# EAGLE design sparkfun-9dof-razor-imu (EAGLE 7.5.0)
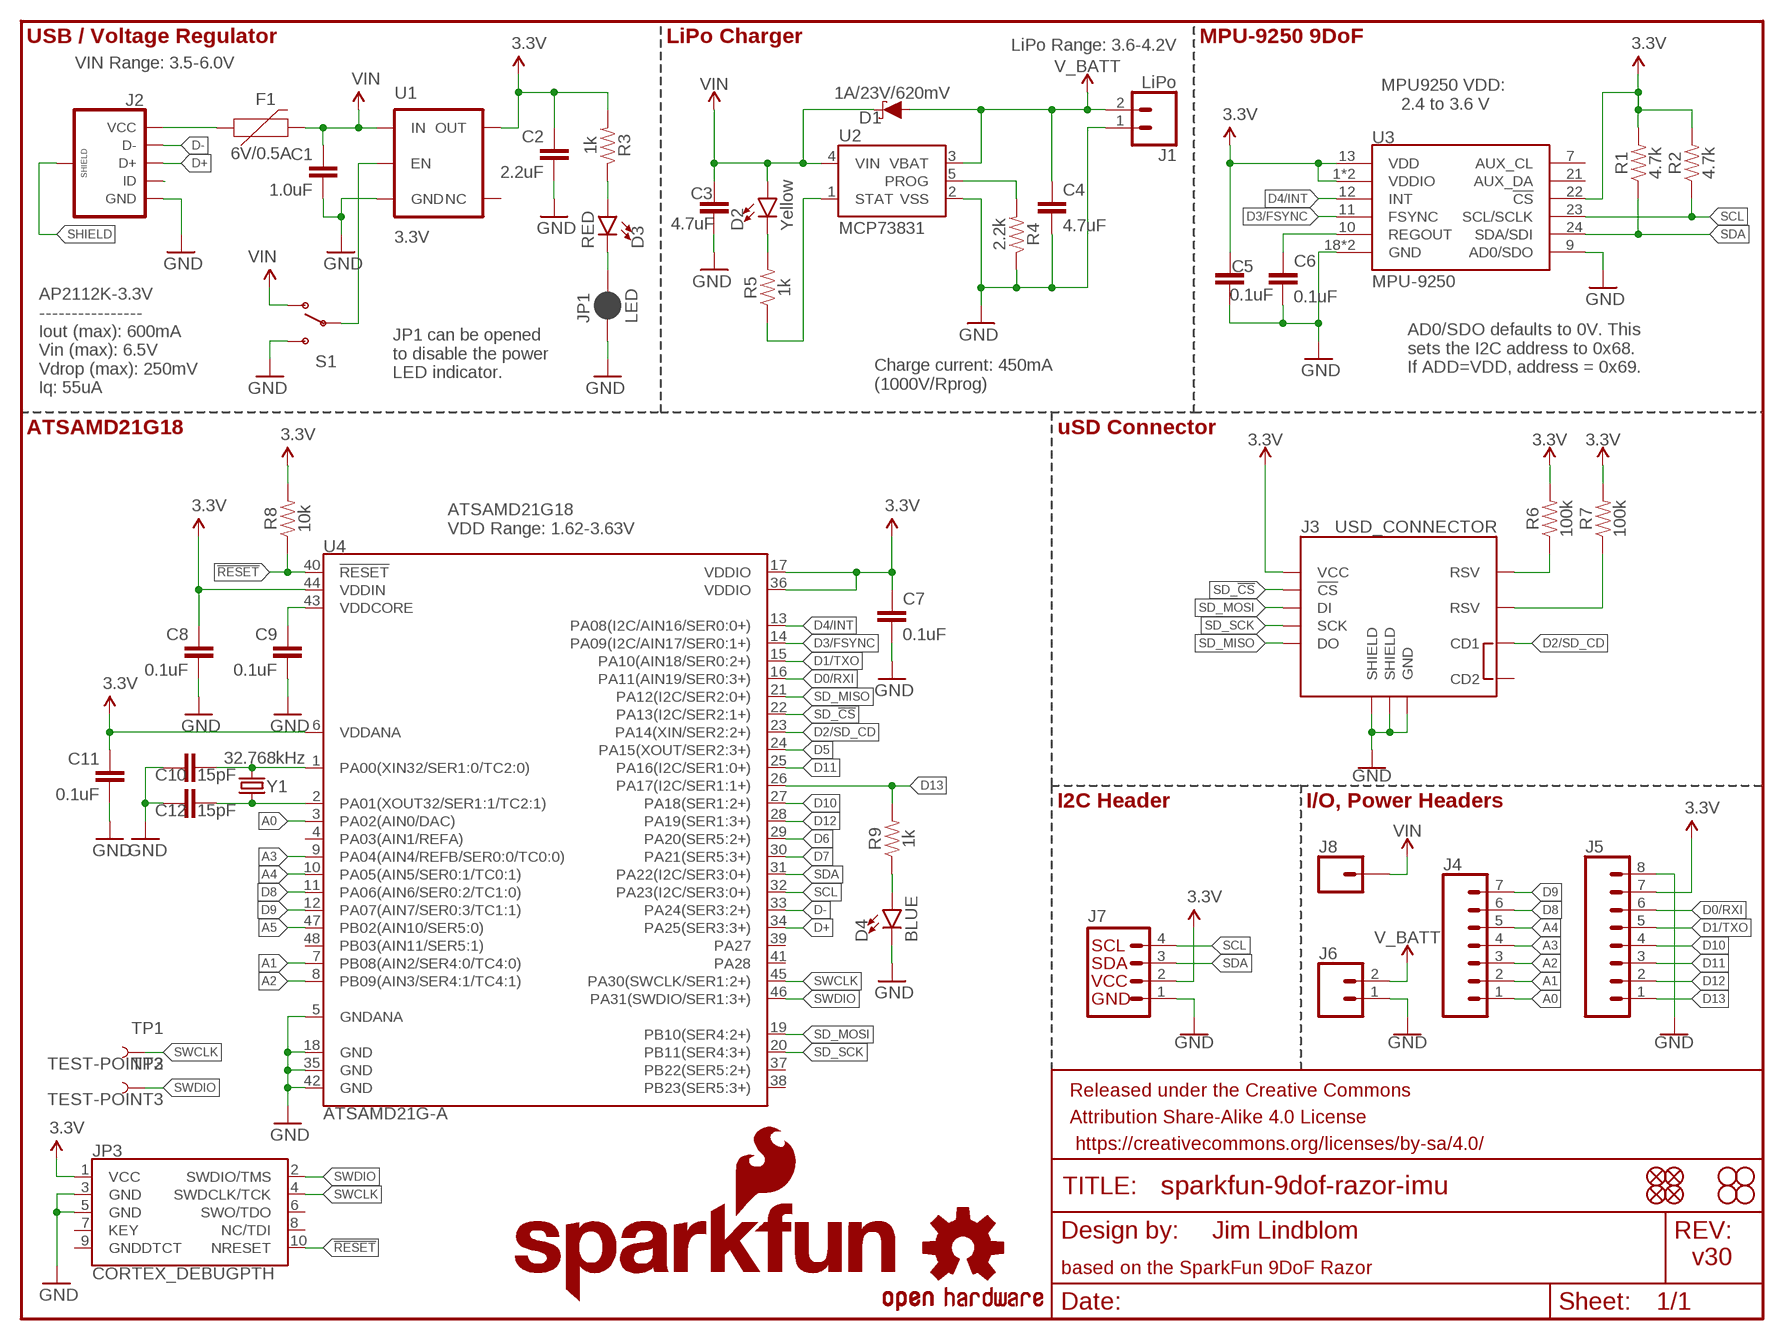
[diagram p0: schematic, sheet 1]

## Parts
C1  1.0uF  1.0UF-0603-16V-10%  [0603]
C2  2.2uF  2.2UF-0603-10V-20%  [0603]
C3  4.7uF  4.7UF0603  [0603]
C4  4.7uF  4.7UF0603  [0603]
C5  0.1uF  0.1UF-0603-25V-(+80/-20%)  [0603]
C6  0.1uF  0.1UF-0603-25V-(+80/-20%)  [0603]
C7  0.1uF  0.1UF-0603-25V-(+80/-20%)  [0603]
C8  0.1uF  0.1UF-0603-25V-(+80/-20%)  [0603]
C9  0.1uF  0.1UF-0603-25V-(+80/-20%)  [0603]
C10  15pF  15PF-0603-50V-5%  [0603]
C11  0.1uF  0.1UF-0603-100V-10%  [0603]
C12  15pF  15PF-0603-50V-5%  [0603]
D1  1A/23V/620mV  DIODE-SCHOTTKY-BAT20J  [SOD-323]
D2  Yellow  LED-YELLOW0603  [LED-0603]
D3  RED  LED-RED0603  [LED-0603]
D4  BLUE  LED-BLUE0603  [LED-0603]
F1  6V/0.5A  PPTC_HALF-AMP  [1206]
FD1  FIDUCIAL1X2  [FIDUCIAL-1X2]
FD2  FIDUCIAL1X2  [FIDUCIAL-1X2]
FD3  FIDUCIAL1X2  [FIDUCIAL-1X2]
FD4  FIDUCIAL1X2  [FIDUCIAL-1X2]
FRAME1  FRAME-LETTER  [CREATIVE_COMMONS]
H1  STAND-OFF  [STAND-OFF]
H2  STAND-OFF  [STAND-OFF]
H3  STAND-OFF  [STAND-OFF]
H4  STAND-OFF  [STAND-OFF]
J1  LiPo  CONN_02-JST-2MM-SMT  [JST-2-SMD]
J2  USB_MICROB_PLUGCONN-11752  [USB-B-MICRO-SMD_V03]
J3  USD_CONNECTOR  [MICRO-SD-SOCKET-PP]
J4  CONN_07  [1X07]
J5  CONN_08"  [1X08]
J6  CONN_02  [1X02]
J7  I2C_STANDARD  [1X04]
J8  CONN_01  [1X01]
JP1  LED  JUMPER-SMT_2_NC_PASTE_NO-SILK  [SMT-JUMPER_2_NC_PASTE_NO-SILK]
JP3  CORTEX_DEBUGPTH  [2X5-PTH-1.27MM]
LOGO1  SFE_LOGO_FLAME.1_INCH  [SFE_LOGO_FLAME_.1]
LOGO2  OSHW-LOGOS  [OSHW-LOGO-S]
LOGO3  SFE_LOGO_NAME.1_INCH  [SFE_LOGO_NAME_.1]
R1  4.7k  4.7KOHM-0603-1/10W-1%  [0603]
R2  4.7k  4.7KOHM-0603-1/10W-1%  [0603]
R3  1k  1KOHM-0603-1/10W-1%  [0603]
R4  2.2k  2.2KOHM-0603-1/10W-1%  [0603]
R5  1k  1KOHM-0603-1/10W-1%  [0603]
R6  100k  100KOHM-0603-1/10W-1%  [0603]
R7  100k  100KOHM-0603-1/10W-1%  [0603]
R8  10k  10KOHM-0603-1/10W-1%  [0603]
R9  1k  1KOHM-0603-1/10W-1%  [0603]
S1  SWITCH-SPDT-SMD-A  [SWITCH-SPST-SMD-A]
TP1  TEST-POINT3  [PAD.03X.03]
TP2  TEST-POINT3  [PAD.03X.03]
U1  3.3V  V_REG_AP2112K-3.3V  [SOT23-5]
U2  MCP73831  [SOT23-5]
U3  MPU-9250  [QFN24-3X3]
U4  ATSAMD21G-A  [TQFP-48]
Y1  32.768kHz  CRYSTAL-32.768KHZSMD-3.2X1.5  [CRYSTAL-SMD-3.2X1.5MM]

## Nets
3.3V: C2.1 C5.1 C7.1 C8.1 C11.1 J3.VCC J5.7 J7.2 JP3.1(VCC) R1.2 R2.2 R3.2 R6.2 R7.2 R8.2 U1.5(OUT) U3.1(VDDIO) U3.8(VDDIO) U3.13(VDD) U3.22(!CS) U4.6(VDDANA) U4.17(VDDIO) U4.36(VDDIO) U4.44(VDDIN)
!RESET: JP3.10(NRESET) R8.1 U4.40(!RESET!)
A0: J4.1 U4.3(PA02(AIN0/DAC))
A1: J4.2 U4.7(PB08(AIN2/SER4:0/TC4:0))
A2: J4.3 U4.8(PB09(AIN3/SER4:1/TC4:1))
A3: J4.4 U4.9(PA04(AIN4/REFB/SER0:0/TC0:0))
A4: J4.5 U4.10(PA05(AIN5/SER0:1/TC0:1))
A5: U4.47(PB02(AIN10/SER5:0))
CHG_LED: R5.1 U2.1(STAT)
D0/RXI: J5.6 U4.16(PA11(AIN19/SER0:3+))
D1/TXO: J5.5 U4.15(PA10(AIN18/SER0:2+))
D2/SD_CD: J3.CD1 U4.23(PA14(XIN/SER2:2+))
D3/FSYNC: U3.11(FSYNC) U4.14(PA09(I2C/AIN17/SER0:1+))
D4/INT: U3.12(INT) U4.13(PA08(I2C/AIN16/SER0:0+))
D5: U4.24(PA15(XOUT/SER2:3+))
D6: U4.29(PA20(SER5:2+))
D7: U4.30(PA21(SER5:3+))
D8: J4.6 U4.11(PA06(AIN6/SER0:2/TC1:0))
D9: J4.7 U4.12(PA07(AIN7/SER0:3/TC1:1))
D10: J5.4 U4.27(PA18(SER1:2+))
D11: J5.3 U4.25(PA16(I2C/SER1:0+))
D12: J5.2 U4.28(PA19(SER1:3+))
D13: J5.1 R9.2 U4.26(PA17(I2C/SER1:1+))
D+: J2.D+ U4.34(PA25(SER3:3+))
D-: J2.D- U4.33(PA24(SER3:2+))
GND: C1.2 C2.2 C3.2 C4.2 C5.2 C6.2 C7.2 C8.2 C9.2 C10.1 C11.2 C12.2 D4.C J1.1 J2.GND J3.GND J3.GND1(SHIELD) J3.GND3(SHIELD) J5.8 J6.1 J7.1 JP1.1 JP3.3(GND) JP3.5(GND) R4.1 S1.3(S) U1.2(GND) U2.2(VSS) U3.9(AD0/SDO) U3.18(GND) U3.20(GND) U4.5(GNDANA) U4.18(GND) U4.35(GND) U4.42(GND)
ID: J2.ID
N$1: F1.1 J2.VBUS(VCC)
N$2: C10.2 U4.1(PA00(XIN32/SER1:0/TC2:0)) Y1.P$2
N$3: D4.A R9.1
N$4: C12.1 U4.2(PA01(XOUT32/SER1:1/TC2:1)) Y1.P$1
N$5: D3.A R3.1
N$7: R4.2 U2.5(PROG)
N$8: J3.RSV1(RSV) R6.1
N$9: J3.RSV2(RSV) R7.1
N$11: D2.C R5.2
N$12: D3.C JP1.2
REGOUT: C6.1 U3.10(REGOUT)
SCL: J7.4 R2.1 U3.23(SCL/SCLK) U4.32(PA23(I2C/SER3:0+))
SD_!CS!: J3.CS(!CS) U4.22(PA13(I2C/SER2:1+))
SD_MISO: J3.DO U4.21(PA12(I2C/SER2:0+))
SD_MOSI: J3.DI U4.19(PB10(SER4:2+))
SD_SCK: J3.SCLK(SCK) U4.20(PB11(SER4:3+))
SDA: J7.3 R1.1 U3.24(SDA/SDI) U4.31(PA22(I2C/SER3:0+))
SHIELD: J2.SHIELD1(SHIELD) J2.SHIELD2(SHIELD) J2.SHIELD3(SHIELD)
SWCLK: JP3.4(SWDCLK/TCK) TP1.P$1 U4.45(PA30(SWCLK/SER1:2+))
SWDIO: JP3.2(SWDIO/TMS) TP2.P$1 U4.46(PA31(SWDIO/SER1:3+))
V_BATT: C4.1 D1.A J1.2 J6.2 U2.3(VBAT)
VDDCORE: C9.1 U4.43(VDDCORE)
VIN: C1.1 C3.1 D1.C D2.A F1.2 J8.1 S1.1(O) U1.1(IN) U2.4(VIN)
VREG_EN: S1.2(P) U1.3(EN)
Unconnected: J3.CD2 JP3.6(SWO/TDO) JP3.7(KEY) JP3.8(NC/TDI) JP3.9(GNDDTCT) U1.4(NC) U3.7(AUX_CL) U3.21(AUX_DA) U4.4(PA03(AIN1/REFA)) U4.37(PB22(SER5:2+)) U4.38(PB23(SER5:3+)) U4.39(PA27) U4.41(PA28) U4.48(PB03(AIN11/SER5:1))

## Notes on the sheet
- USB / Voltage Regulator | LiPo Charger | MPU-9250 9DoF
- LiPo Range: 3.6-4.2V
- VIN Range: 3.5-6.0V
- MPU9250 VDD:
   2.4 to 3.6 V
- AP2112K-3.3V
  ----------------
  Iout (max): 600mA 
  Vin (max): 6.5V
  Vdrop (max): 250mV
  Iq: 55uA
- AD0/SDO defaults to 0V. This 
  sets the I2C address to 0x68.
  If ADD=VDD, address = 0x69.
- JP1 can be opened
  to disable the power
  LED indicator.
- Charge current: 450mA
  (1000V/Rprog)
- ATSAMD21G18 | uSD Connector
- ATSAMD21G18
  VDD Range: 1.62-3.63V
- I2C Header | I/O, Power Headers
- Jim Lindblom
- v30
- based on the SparkFun 9DoF Razor

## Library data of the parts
C1 = SparkFun-Capacitors:1.0UF: 1µF ceramic capacitors; PROD_ID: CAP-00868
C2 = SparkFun-Capacitors:2.2UF: 2.2µF ceramic capacitors; PROD_ID: CAP-07888
C3 C4 = SparkFun-Capacitors:4.7UF: 4.7µF ceramic capacitors; PROD_ID: CAP-08280
C5-C9 = SparkFun-Capacitors:0.1UF: 0.1µF ceramic capacitors; PROD_ID: CAP-00810
C10 C12 = SparkFun-Capacitors:15PF: 15pF ceramic capacitors; PROD_ID: CAP-07881
C11 = SparkFun-Capacitors:0.1UF: 0.1µF ceramic capacitors; PROD_ID: CAP-08390
D1 = SparkFun-DiscreteSemi:DIODE-SCHOTTKY: Schottky diode; PROD_ID: DIO-11623
D2 = SparkFun-LED:LED-YELLOW: Yellow SMD LED; PROD_ID: DIO-09003
D3 = SparkFun-LED:LED-RED: Red SMD LED; PROD_ID: DIO-00819
D4 = SparkFun-LED:LED-BLUE: Blue SMD LED; PROD_ID: DIO-08575
F1 = SparkFun-Fuses:PPTC: Resettable Fuse PPTC; PROD_ID: RES-08585
FD1-FD4 = SparkFun-Aesthetics:FIDUCIAL: Fiducial Alignment Points
FRAME1 = SparkFun-Aesthetics:FRAME-LETTER: Schematic Frame - Letter
H1-H4 = SparkFun-Electromechanical:STAND-OFF: #4 Stand Off
J1 = SparkFun-Connectors:CONN_02: Multi connection point. Often used as Generic Header-pin footprint for 0.1 inch spaced/style header connections; PROD_ID: CONN-11443
J2 = SparkFun-Connectors:USB_MICROB_PLUG: USB Micro-B connectors Some male, some female. Watch your step!; PROD_ID: CONN-11752
J3 = SparkFun-Connectors:USD_CONNECTOR: microSD Socket Push-push type µSD socket. Footprint production proven. Symbol has new and improved layout and naming accuracy. SparkFun Electronics SKU : PRT-00127. tDoc lines correctly indicate media card edge positions when inserting (unlocked, locked, depressed). NOTE: CD1 and CD2 are connected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; PROD_ID: CONN-07820
J4 = SparkFun-Connectors:CONN_07: Multi connection point. Often used as Generic Header-pin footprint for 0.1 inch spaced/style header connections On any of the 0.1 inch spaced packages, you can populate with these: Break Away Headers - Straight (PRT-00116) Break Away Male Headers - Right Angle (PRT-00553) Female Headers (PRT-00115)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
J5 = SparkFun-Connectors:CONN_08: Multi connection point. Often used as Generic Header-pin footprint for 0.1 inch spaced/style header connections On any of the 0.1 inch spaced packages, you can populate with these: Break Away Headers - Straight (PRT-00116) Break Away Male Headers - Right Angle (PRT-00553) Female Headers (PRT-00115)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
J6 = SparkFun-Connectors:CONN_02: Multi connection point. Often used as Generic Header-pin footprint for 0.1 inch spaced/style header connections
J7 = SparkFun-Connectors:I2C_STANDARD: SparkFun has standardized on a pinout for all I2C based sensor breakouts. This pinout allows I2C boards to be plugged directly into the headers on Arduino Uno compatible boards, and to be daisy chained easily.
J8 = SparkFun-Connectors:CONN_01: Single connection point. Often used as Generic Header-pin footprint for 0.1 inch spaced/style header connections
JP1 = SparkFun-Jumpers:JUMPER-SMT_2_NC_PASTE: Normally closed solder jumper
JP3 = samd21-temp:CORTEX_DEBUG: Cortex Debug Connector Datasheet
LOGO1 = SparkFun-Aesthetics:SFE_LOGO_FLAME: SFE Logo, flame only
LOGO2 = SparkFun-Aesthetics:OSHW-LOGO: Open Source Hardware Logo
LOGO3 = SparkFun-Aesthetics:SFE_LOGO_NAME: SparkFun Font Logo
R1 R2 = SparkFun-Resistors:4.7KOHM: 4.7kΩ resistor; PROD_ID: RES-07857
R3 R5 R9 = SparkFun-Resistors:1KOHM: 1kΩ resistor; PROD_ID: RES-07856
R4 = SparkFun-Resistors:2.2KOHM: 2.2kΩ resistor; PROD_ID: RES-08272
R6 R7 = SparkFun-Resistors:100KOHM: 100kΩ resistor; PROD_ID: RES-07828
R8 = SparkFun-Resistors:10KOHM: 10kΩ resistor; PROD_ID: RES-00824
S1 = SparkFun-Electromechanical:SWITCH-SPDT: SPDT Switch Simple slide switch, Spark Fun Electronics SKU : COM-00102 DPDT SMT slide switch, AYZ0202, SWCH-08179; PROD_ID: SWCH-10651
TP1 TP2 = SparkFun-Connectors:TEST-POINT: Bare copper test points for troubleshooting or ICT
U1 = SparkFun-IC-Power:V_REG_AP2112: AP2112 - 600mA CMOS LDO Regulator w/ Enable The AP2112 is CMOS process low dropout linear regulator with enable function, the regulator delivers a guaranteed 600mA (min.) continuous load current. Features Output Voltage Accuracy: ±1.5% Output Current: 600mA (Min.) Foldback Short Current Protection: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; PROD_ID: VREG-12457
U2 = SparkFun-IC-Power:MCP73831: Miniature single cell, fully integrated Li-Ion, Li-polymer charge management controller http://ww1.microchip.com/downloads/en/DeviceDoc/20001984g.pdf IC-09995; PROD_ID: IC-09995
U3 = 9dof-devboard-temp:MPU-9250: NC pin 19. 2-6 & 14-17 not internally connected. May be used for PCB trace routing.; PROD_ID: IC-13192
U4 = SparkFun-IC-Microcontroller:ATSAMD21G: Atmel SAMD21G SMART ARM-Based Microcontroller The Atmel ® | SMART ™ SAM D21 is a series of low-power microcontrollers using the 32-bit ARM ® Cortex ® -M0+ processor, and ranging from 32- to 64-pins with up to 256KB Flash and 32KB of SRAM. The SAM D21 devices operate at a maximum frequency of 48MHz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; PROD_ID: IC-13064
Y1 = SparkFun-Clocks:CRYSTAL-32.768KHZ: 32.768kHz Crystal; PROD_ID: XTAL-13062

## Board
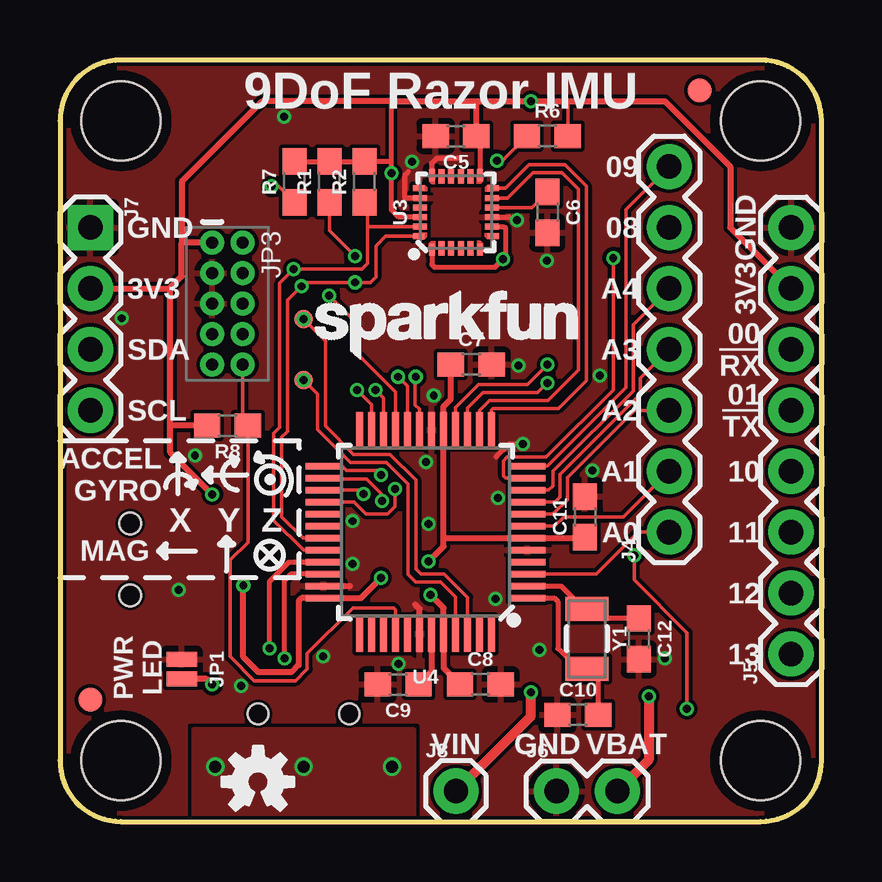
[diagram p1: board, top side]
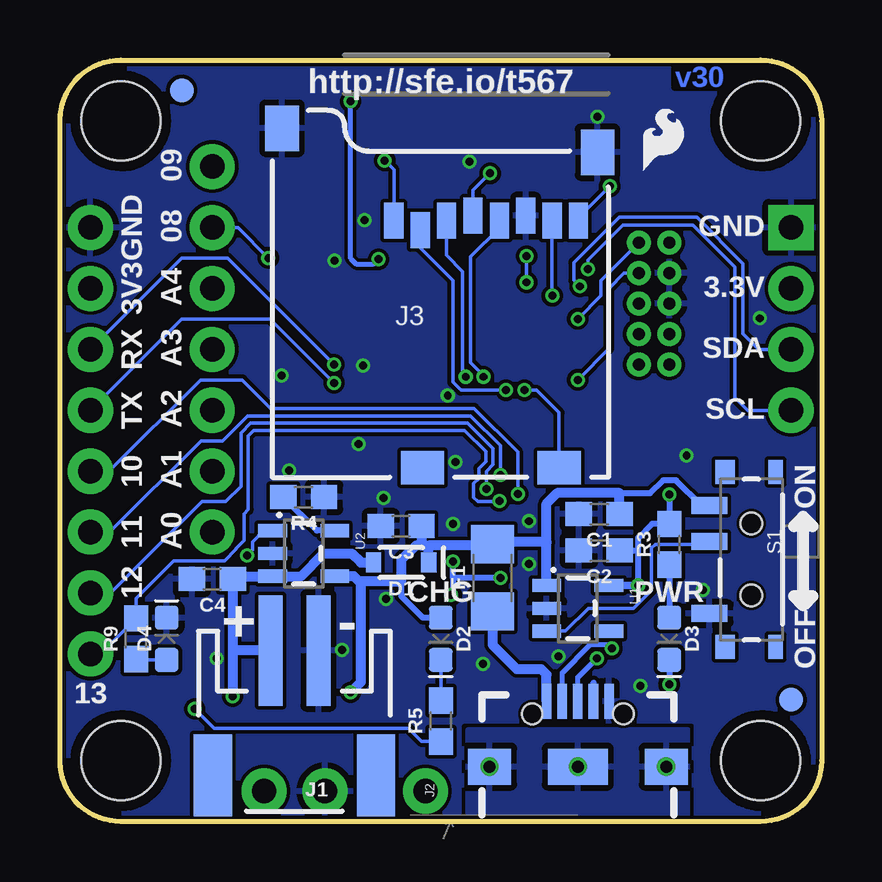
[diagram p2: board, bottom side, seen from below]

Size 31.75 x 31.75 mm. Coordinates in mm from the lower left corner, seen from the top.
Outline: 2.54,0 29.21,0 arc90 31.75,2.54 31.75,29.21 arc90 29.21,31.75 2.54,31.75 arc90 0,29.21 0,2.54 arc90 2.54,0
Copper layers (1*16): Top 0.035mm / dielectric 1.5mm / Bottom 0.035mm
Design rules "SparkFun-2-layer-FAB-LIMIT *": minimum track width 4mil, minimum drill 6mil, track to track 6mil, track to pad 6mil, pad to pad 6mil, via to via 6mil, smd to smd 6mil, copper to edge 4mil, drill to drill 4mil, minimum pad ring 5mil, minimum via ring 5mil, stop-mask expansion 4mil, vias tented up to drill 25mil, thermal gap 10mil

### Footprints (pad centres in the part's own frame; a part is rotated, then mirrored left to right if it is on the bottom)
0603 = smd 1.1 x 1: 1 -0.85,0; 2 0.85,0
SOD-323 = smd 0.63 x 0.83: A 1.15,0; C -1.15,0
LED-0603 = smd 1 x 1: A -0.877,0; C 0.877,0
1206 = smd 1.6 x 1.8: 1 -1.4,0; 2 1.4,0
FIDUCIAL-1X2 = smd 1 x 1: 1 0,0
STAND-OFF = hole 3.302: 0,0
JST-2-SMD = smd 1 x 4.6: 1 -1,-3.7; 2 1,-3.7 | smd 1.6 x 3.4: NC1 -3.4,1.5; NC2 3.4,1.5
USB-B-MICRO-SMD_V03 = smd 1.45 x 0.4: D+ 2.725,0; D- 2.725,0.65; GND 2.725,-1.3; ID 2.725,-0.65; VBUS 2.725,1.3 | smd 1.5 x 1.8: SHIELD1 0,3.685; SHIELD2 0,-3.685 | smd 1.5 x 2.5: SHIELD3 0,0 | hole 0.85: 2.2,1.9; 2.2,-1.9
MICRO-SD-SOCKET-PP = smd 1.8 x 1.4: CD1 -2.05,0.4; CD2 -7.75,0.4 | smd 0.8 x 1.5: CS -7.84,10.3; DI -6.74,10.7; DO -2.34,10.7; GND -3.44,10.9; RSV1 -8.94,10.7; RSV2 -1.24,10.7; SCLK -4.54,10.7; VCC -5.64,10.9 | smd 1.4 x 1.9: GND1 -13.6,14.55; GND3 -0.45,13.55
1X07 = drill 1.016 pad 1.88: 1 0,0; 2 2.54,0; 3 5.08,0; 4 7.62,0; 5 10.16,0; 6 12.7,0; 7 15.24,0
1X08 = drill 1.016 pad 1.88: 1 0,0; 2 2.54,0; 3 5.08,0; 4 7.62,0; 5 10.16,0; 6 12.7,0; 7 15.24,0; 8 17.78,0
1X02 = drill 1.016 pad 1.88: 1 0,0; 2 2.54,0
1X04 = drill 1.016 pad 1.88 square: 1 0,0 | drill 1.016 pad 1.88: 2 2.54,0; 3 5.08,0; 4 7.62,0
1X01 = drill 1.016 pad 1.88: 1 0,0
SMT-JUMPER_2_NC_PASTE_NO-SILK = smd 0.635 x 1.27: 1 -0.406,0; 2 0.406,0
2X5-PTH-1.27MM = drill 0.508 pad 1: 1 -2.54,-0.635; 2 -2.54,0.635; 3 -1.27,-0.635; 4 -1.27,0.635; 5 0,-0.635; 6 0,0.635; 7 1.27,-0.635; 8 1.27,0.635; 9 2.54,-0.635; 10 2.54,0.635
SWITCH-SPST-SMD-A = smd 0.7 x 1.5: 1 -2.25,-1.75; 2 -0.75,-1.75; 3 2.25,-1.75 | smd 1 x 0.6: GND1 -3.65,1; GND3 3.65,1 | smd 1 x 0.8: GND2 -3.65,-1.1; GND4 3.65,-1.1 | hole 0.9: -1.5,0; 1.5,0
PAD.03X.03 = smd 0.762 x 0.762: P$1 0,0
SOT23-5 = smd 0.55 x 1.2: 1 -0.95,-1.3; 2 0,-1.3; 3 0.95,-1.3; 4 0.95,1.3; 5 -0.95,1.3
QFN24-3X3 = smd 0.495 x 0.25: 1 -1.552,1; 6 -1.552,-1; 13 1.552,-1; 18 1.552,1 | smd 0.6 x 0.25: 2 -1.5,0.6; 3 -1.5,0.2; 4 -1.5,-0.2; 5 -1.5,-0.6; 14 1.5,-0.6; 15 1.5,-0.2; 16 1.5,0.2; 17 1.5,0.6 | smd 0.25 x 0.495: 7 -1,-1.552; 12 1,-1.552; 19 1,1.552; 24 -1,1.552 | smd 0.25 x 0.6: 8 -0.6,-1.5; 9 -0.2,-1.5; 10 0.2,-1.5; 11 0.6,-1.5; 20 0.6,1.5; 21 0.2,1.5; 22 -0.2,1.5; 23 -0.6,1.5
TQFP-48 = smd 1.5 x 0.28: 1 -4.25,2.75; 2 -4.25,2.25; 3 -4.25,1.75; 4 -4.25,1.25; 5 -4.25,0.75; 6 -4.25,0.25; 7 -4.25,-0.25; 8 -4.25,-0.75; 9 -4.25,-1.25; 10 -4.25,-1.75; 11 -4.25,-2.25; 12 -4.25,-2.75; 25 4.25,-2.75; 26 4.25,-2.25; 27 4.25,-1.75; 28 4.25,-1.25; 29 4.25,-0.75; 30 4.25,-0.25; 31 4.25,0.25; 32 4.25,0.75; 33 4.25,1.25; 34 4.25,1.75; 35 4.25,2.25; 36 4.25,2.75 | smd 0.28 x 1.5: 13 -2.75,-4.25; 14 -2.25,-4.25; 15 -1.75,-4.25; 16 -1.25,-4.25; 17 -0.75,-4.25; 18 -0.25,-4.25; 19 0.25,-4.25; 20 0.75,-4.25; 21 1.25,-4.25; 22 1.75,-4.25; 23 2.25,-4.25; 24 2.75,-4.25; 37 2.75,4.25; 38 2.25,4.25; 39 1.75,4.25; 40 1.25,4.25; 41 0.75,4.25; 42 0.25,4.25; 43 -0.25,4.25; 44 -0.75,4.25; 45 -1.25,4.25; 46 -1.75,4.25; 47 -2.25,4.25; 48 -2.75,4.25
CRYSTAL-SMD-3.2X1.5MM = smd 1 x 1.8: P$1 -1.25,0; P$2 1.25,0

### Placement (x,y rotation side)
C1  9.27,12.83 180 bottom
C2  9.27,11.3 180 bottom
C3  17.53,12.32 180 bottom
C4  25.4,10.11 180 bottom
C5  16.51,28.57 180 top
C6  20.32,25.4 270 top
C7  17.14,19.05 0 top
C8  17.53,5.71 0 top
C9  14.1,5.71 180 top
C10  21.59,4.45 0 top
C11  21.89,12.7 90 top
C12  24.13,7.62 270 top
D1  17.53,10.79 180 bottom
D2  15.88,7.62 270 bottom
D3  6.35,7.62 270 bottom
D4  27.3,7.62 90 bottom
F1  13.72,10.16 90 bottom
FD1  1.27,5.08 0 bottom
FD2  26.67,30.48 0 top
FD3  26.67,30.48 0 bottom
FD4  1.27,5.08 0 top
FRAME1  not placed on the board
H1  29.21,2.54 0 top
H2  2.54,2.54 0 top
H3  29.21,29.21 0 top
H4  2.54,29.21 0 top
J1  21.97,3.43 180 bottom
J2  10.16,2.29 90 bottom
J3  8.89,14.35 0 bottom
J4  25.4,12.06 90 top
J5  30.48,6.99 90 top
J6  20.7,1.27 0 top
J7  1.27,24.77 270 top
J8  16.51,1.27 0 top
JP1  5.08,6.35 270 top
JP3  6.99,21.59 270 top
LOGO1  7.75,26.8 0 bottom
LOGO2  8.26,1.65 0 top
LOGO3  10.16,18.8 0 top
R1  11.24,26.67 90 top
R2  12.7,26.67 90 top
R3  6.35,11.56 90 bottom
R4  21.59,13.53 180 bottom
R5  15.88,4.19 90 bottom
R6  20.32,28.57 0 top
R7  9.78,26.67 90 top
R8  6.99,16.51 180 top
R9  28.57,7.62 90 bottom
S1  2.92,10.92 270 bottom
TP1  10.16,18.41 0 top
TP2  10.16,20.95 0 top
U1  10.16,8.89 270 bottom
U2  21.59,11.18 270 bottom
U3  16.51,25.4 90 top
U4  15.24,12.06 180 top
Y1  21.97,7.62 270 top

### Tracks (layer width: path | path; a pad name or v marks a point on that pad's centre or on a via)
3.3V  (via drill 0.33)
  Top 0.152: R6.2 21.17,30.02 21.59,30.02
  Top 0.203: U3.22 14.12,25.2 13.82,25.5 v13.82,27.03 13.82,27.53 | R7.2 R1.2 R2.2 12.71,27.53 13.82,27.53 | C5.1 17.51,28.43 U3.13 | 13.82,27.53 13.82,30.02 | U3.8 18.51,24.8 18.59,24.71 18.59,23.57 v18.47,23.44 18.14,23.11 15.62,23.11 15.51,23.23 U3.1
  Top 0.254: 15.99,11.81 U4.17 15.99,17.31 16.3,17.62 C7.1 15.99,19.05 | v7.64,9.84 7.64,6.86 8.28,6.22 9.65,6.22 9.96,6.53 9.96,9.2 10.08,9.31 U4.36 12.54,9.31 v13.39,10.16 | 5.08,24.13 5.08,26.67 8.43,30.02 13.82,30.02 17.36,30.02 | JP3.1 5.08,24.13 | 17.36,30.02 v19.63,30.02 21.59,30.02 25.22,30.02 27.94,27.3 27.94,24.77 J5.7 | C5.1 17.36,30.02 | 15.99,11.81 U4.6 21.86,11.81 C11.1 | v15.37,10.85 15.99,11.47 15.99,11.81 | v15.44,9.44 15.57,9.31 15.58,9.31 15.99,8.9 U4.44 15.99,6.4 C8.1 | 5.08,24.13 5.08,22.73 4.6,22.25 4.6,22.23 | 4.6,16.51 4.6,15.39 v6.35,13.64 | 4.6,16.51 4.6,22.23 | J7.2 4.6,22.23 | R8.2 4.6,16.51
  Bottom 0.152: J3.VCC 14.53,26.31 v13.82,27.03
  Bottom 0.203: v19.63,30.02 19.63,23.47 19.41,23.24 18.67,23.24 v18.47,23.44
  Bottom 0.254: v6.35,13.64 R3.2 7.06,12.41 7.64,11.82 7.64,11.3 | v13.39,10.16 15.37,10.16 | 15.37,10.16 v15.37,10.85 | v7.64,9.84 7.64,11.3 | C2.1 7.64,11.3 | 15.37,10.16 15.37,9.52 v15.44,9.44
  Bottom 0.305: U1.5 v7.64,9.84
!RESET
  Top 0.152: U4.40 13.99,8.82 13.9,8.91 12.21,8.91 10.31,7.01 10.31,6.36 9.81,5.87 8.1,5.87 7.09,6.88 7.09,10.9 7.83,11.64 R8.1 7.62,16.73 JP3.10
A0
  Top 0.152: J4.1 24.11,12.06 22.36,10.31 U4.3
A1
  Top 0.152: U4.7 20.62,12.31 21.01,12.7 23.5,12.7 J4.2
A2
  Top 0.152: U4.8 20.56,12.81 21.16,13.41 21.16,14.35 23.95,17.14 J4.3
A3
  Top 0.152: U4.9 20.63,13.31 20.85,13.54 20.85,14.48 24.21,17.83 24.21,18.49 J4.4
A4
  Top 0.152: U4.10 20.37,13.81 20.55,13.99 20.55,14.61 23.9,17.96 23.9,20.73 J4.5
CHG_LED  (via drill 0.33)
  Top 0.152: v26.14,4.7 26.14,7.87 23.94,10.07 v23.94,11.1
  Bottom 0.152: v26.14,4.7 25.32,3.89 17.22,3.89 16.68,3.34 R5.1 | v23.94,11.1 23.72,11.32 23.72,11.66 23.26,12.13 U2.1
D0/RXI  (via drill 0.33)
  Top 0.152: U4.16 16.49,17.25 17.45,18.21 19.48,18.21 v20.32,19.05
  Bottom 0.152: v20.32,19.05 24.77,23.5 26.67,23.5 J5.6
D1/TXO  (via drill 0.33)
  Top 0.152: U4.15 16.99,17.24 17.63,17.88 19.91,17.88 v20.32,18.29
  Bottom 0.152: v20.32,18.29 22.99,20.95 26.67,20.95 J5.5
D2/SD_CD  (via drill 0.33)
  Top 0.152: U4.23 12.99,17.38 v12.39,17.98
  Bottom 0.152: J3.CD1 10.94,17.04 11.88,17.98 v12.39,17.98
D3/FSYNC
  Top 0.152: U4.14 17.49,17.13 17.91,17.55 20.34,17.55 21.61,18.82 21.61,26.36 20.93,27.05 19.71,27.05 18.66,26 U3.11
D4/INT
  Top 0.152: U4.13 17.99,17.15 18.06,17.22 20.78,17.22 21.95,18.39 21.95,26.49 21.06,27.38 19.56,27.38 18.58,26.4 U3.12
D8  (via drill 0.33)
  Top 0.152: U4.11 18.58,14.31 18.49,14.4 18.49,15.04 18.64,15.19 20.27,15.19 23.06,17.98 v23.06,23.5
  Bottom 0.152: J4.6 24.33,24.77 v23.06,23.5
D9
  Top 0.152: U4.12 20.33,14.81 23.6,18.09 23.6,25.5 J4.7
D10  (via drill 0.33)
  Top 0.152: U4.27 12.5,13.81 v12.66,13.65
  Bottom 0.152: v12.66,13.65 12.66,15.4 14.48,17.22 22.96,17.22 24.16,18.41 25.88,18.41 29.69,14.61 J5.4
D11  (via drill 0.33)
  Top 0.152: U4.25 11.75,14.81 11.94,14.63 13.2,14.63 v13.39,14.44
  Bottom 0.152: J5.3 29.67,12.06 25.86,15.88 24.97,15.88 23.93,16.92 14.63,16.92 13.39,15.67 v13.39,14.44
D12  (via drill 0.33)
  Top 0.152: v13.97,13.87 13.97,13.14 13.66,12.83 12.75,12.83 12.26,13.31 U4.28
  Bottom 0.152: J5.2 29.64,9.53 25.83,13.34 24.84,13.34 24.21,13.97 24.21,16.2 23.8,16.61 14.76,16.61 13.69,15.54 13.69,14.88 13.97,14.6 v13.97,13.87
D13  (via drill 0.33)
  Top 0.152: v13.43,13.36 13.43,13.64 12.79,14.29 11.02,14.29 U4.26
  Bottom 0.152: v13.43,13.36 13.46,13.34 14.33,13.34 14.5,13.51 14.5,14.08 14.29,14.3 14.29,14.72 13.99,15.01 13.99,15.42 14.88,16.31 23.67,16.31 23.9,16.08 23.9,13.01 24.08,12.83 24.08,11.71 24.4,11.39 24.4,11.36 24.89,10.87 27,10.87 28.57,9.3 R9.2 30.06,6.99 J5.1
D+  (via drill 0.33)
  Top 0.203: v9.37,6.81 9.37,10.06 9.63,10.31 U4.34
  Bottom 0.203: J2.D+ 10.16,6.02 v9.37,6.81
D-  (via drill 0.33)
  Top 0.203: v8.74,7.21 8.74,10.01 9.54,10.81 U4.33
  Bottom 0.203: v8.74,7.21 8.89,7.37 9.65,7.37 10.81,6.21 J2.D-
GND  (via drill 0.33)
  Top 0.203: U3.9 18.74,25.2 | U3.18 15.51,27.45 15.72,27.66 16.59,27.66 | U3.20 14.39,26 14.38,26.01 14.38,26.95 14.53,27.1 | 18.19,15.21 18.72,15.75 v19.3,15.75
  Top 0.254: U4.42 14.99,8.86 14.81,9.04 | U4.35 12.08,9.81
  other vias: 12.19,10.74 15.37,12.41 14.68,27.51 19.05,25.07 19.99,7.16 9.35,29.39 18.15,9.28 20.29,23.39 15.25,14.99 2.58,20.98 5.63,15.27 12.19,12.52 22.2,14.64 18.26,13.49 7.54,5.66 10.97,6.88 4.94,9.66 14.12,6.57 25.22,6.79 15.58,17.77 19.11,19.01 22.5,18.59
  pour Bottom (isolate 0.152, rank 6): 31.75,0 31.75,31.75 0,31.75 0,0
  pour Top (isolate 0.152, rank 6): 0,0 0,31.75 31.75,31.75 31.75,0
ID
  Bottom 0.254: J2.ID 9.51,5.79
N$1
  Bottom 0.406: F1.1 13.72,7.37 12.7,6.35 11.68,6.35 11.46,6.13 J2.VBUS
N$2
  Top 0.203: U4.1 20.61,9.31 20.75,9.17 20.75,7.21 21.59,6.37 Y1.P$2 22.44,5.9 C10.2
N$3
  Bottom 0.152: D4.A 28.55,6.74 R9.1
N$4
  Top 0.203: U4.2 20.89,9.81 21.84,8.87 Y1.P$1 22.37,8.47 C12.1
N$5
  Bottom 0.254: R3.1 D3.A
N$7
  Bottom 0.254: U2.5 21.04,12.13 R4.2
N$8  (via drill 0.33)
  Top 0.152: R6.1 18.45,27.56 v18.21,27.56
  Bottom 0.152: J3.RSV1 17.83,27.18 v18.21,27.56
N$9  (via drill 0.33)
  Top 0.152: R7.1 9.11,26.49 v8.83,26.49
  Bottom 0.152: J3.RSV2 10.13,25.18 v8.83,26.49
N$11
  Bottom 0.152: R5.2 D2.C
N$12  (via drill 0.33)
  Top 0.254: v6.35,5.71 6.12,5.94 JP1.2
  Bottom 0.254: D3.C v6.35,5.71
REGOUT
  Top 0.152: U3.10 19.67,25.6 C6.1
SCL  (via drill 0.33)
  Top 0.152: U4.32 10.15,11.31 8.91,12.55 8.91,16.18 9.16,16.42 9.16,22.44 v9.74,23.02 12.59,23.02 12.83,23.27 12.83,24.8 | R2.1 12.7,25.71 12.83,25.59 12.83,24.8 | 12.83,24.8 U3.23
  Bottom 0.152: v9.74,23.02 9.74,23.41 8.28,24.87 5.36,24.87 3.61,23.11 3.61,17.68 3.07,17.14 J7.4
SD_!CS!  (via drill 0.33)
  Top 0.152: U4.22 13.49,17.65 v13.16,17.98
  Bottom 0.152: v13.16,17.98 15.04,17.98 15.37,18.31 15.37,22.55 16.73,23.92 J3.CS
SD_MISO  (via drill 0.33)
  Top 0.152: U4.21 13.99,17.91 12.37,19.53 12.37,20.78 v11.23,21.92
  Bottom 0.152: v11.23,21.92 J3.DO
SD_MOSI  (via drill 0.33)
  Top 0.152: U4.19 14.99,17.19 14.81,17.37 14.81,18.52 v14.83,18.54
  Bottom 0.152: v14.83,18.54 14.96,18.67 14.96,22.94 15.63,23.61 J3.DI
SD_SCK  (via drill 0.33)
  Top 0.152: U4.20 14.49,18.15 v14.1,18.54
  Bottom 0.152: v14.1,18.54 14.1,18.59 14.63,19.13 14.63,23.55 13.43,24.75 J3.SCLK
SDA  (via drill 0.33)
  Top 0.152: U4.31 10.13,11.81 9.25,12.7 9.25,16.03 9.49,16.27 9.49,21.73 v10.07,22.31 10.24,22.48 v12.29,22.48 12.95,22.48 13.17,22.7 13.17,23.99 13.58,24.4 U3.24 | R1.1 11.24,24.62 v12.29,23.57
  Bottom 0.152: J7.3 2.62,19.68 3.28,20.34 3.28,23.27 5.21,25.2 8.43,25.2 10.32,23.3 10.32,22.57 v10.07,22.31 | v12.29,22.48 v12.29,23.57
SHIELD  (via drill 0.51)
  other vias: 6.47,2.29 13.85,2.29 10.16,2.29
  pour Top (isolate 0.152): 5.59,3.81 5.59,0 14.73,0 14.73,3.81
  pour Bottom (isolate 0.152): 5.59,0 5.59,3.81 14.73,3.81 14.73,0
SWCLK  (via drill 0.33)
  Top 0.152: U4.45 16.49,9.37 15.86,9.99 14.82,9.99 14.51,10.31 14.51,14.08 13.61,14.98 12.11,14.98 10.74,16.34 10.74,17.83 TP1.P$1
  Bottom 0.152: JP3.4 8.23,22.86 8.87,22.23 8.87,19.71 TP1.P$1
  other vias: 10.16,18.41
SWDIO  (via drill 0.33)
  Top 0.152: U4.46 16.99,9.35 16.02,10.32 15.05,10.32 14.84,10.54 14.84,14.23 13.76,15.31 12.24,15.31 11.07,16.48 11.07,20.04 TP2.P$1
  Bottom 0.152: JP3.2 9.2,22.55 9.2,21.92 TP2.P$1
  other vias: 10.16,20.95
V_BATT  (via drill 0.33)
  Top 0.406: v24.55,5.22 24.55,2.58 J6.2
  Bottom 0.406: J1.2 24.55,7.13 | D1.A 19.2,10.79 19.58,11.18 20.75,11.18 21.7,10.23 U2.3 24.43,10.23 C4.1 24.55,7.13 | 24.55,7.13 v24.55,5.22
VDDCORE
  Top 0.254: U4.43 15.49,6.26 C9.1
VIN  (via drill 0.33)
  Top 0.406: J8.1 19.63,4.39 v19.63,5.38
  Bottom 0.254: 17.93,9.92 17.93,10.01 | D2.A 16.62,8.5 17.53,9.4 17.53,10.01 | 8.42,13.69 7.14,13.69 6.6,14.22 6.07,14.22 5.02,13.17 S1.1
  Bottom 0.406: U1.1 11.46,11.65 | 11.46,11.65 11.46,13.25 11.02,13.69 8.42,13.69 C1.1 | 16.38,11.51 13.77,11.51 F1.2 13.62,11.65 11.46,11.65 | 16.68,11.51 16.92,11.51 17.53,10.9 17.53,10.01 17.93,10.01 19.2,10.01 | 19.2,10.01 19.28,10.01 19.5,10.23 U2.4 | C3.1 16.68,11.51 | 16.68,11.51 16.38,11.51 | D1.C 16.38,11.51 | v19.63,5.38 19.2,5.82 19.2,10.01
VREG_EN
  Bottom 0.152: S1.2 4.79,11.56 6.93,11.56 7.09,11.4 7.09,9.64 7.84,8.89 9.73,8.89 10.68,7.94 U1.3

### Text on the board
Bottom: v30
tPlace: 9DoF Razor IMU | 09 | GND | 08 | GND | 3V3 | A4 | 3V3 | SDA | A3 | 00 / !RX | SCL | A2 | 01 / !TX | A1 | 10 | ACCEL / GYRO | X | Y | Z | A0 | 11 | MAG | 12 | 13 | PWR / LED | VIN | GND | VBAT
bPlace: http://sfe.io/t567 | 09 | GND | 08 | GND | 3.3V | A4 | 3V3 | SDA | A3 | RX | SCL | A2 | TX | A1 | 10 | ON | A0 | 11 | 12 | PWR | CHG | OFF | - | + | 13
Measures: Units in inches
tDocu: Jim Lindblom

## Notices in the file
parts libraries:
SparkFun-Aesthetics: Licensing: Creative Commons ShareAlike 4.0 International - https://creativecommons.org/licenses/by-sa/4.0
SparkFun-Aesthetics: Released under the Creative Commons Attribution Share-Alike 4.0 License
SparkFun-Aesthetics: https://creativecommons.org/licenses/by-sa/4.0
